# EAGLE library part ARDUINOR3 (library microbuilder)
This is a new object for the new Arduino R3 - with extra pins that you may want to use (such as IOref, and duplicated A4/A5
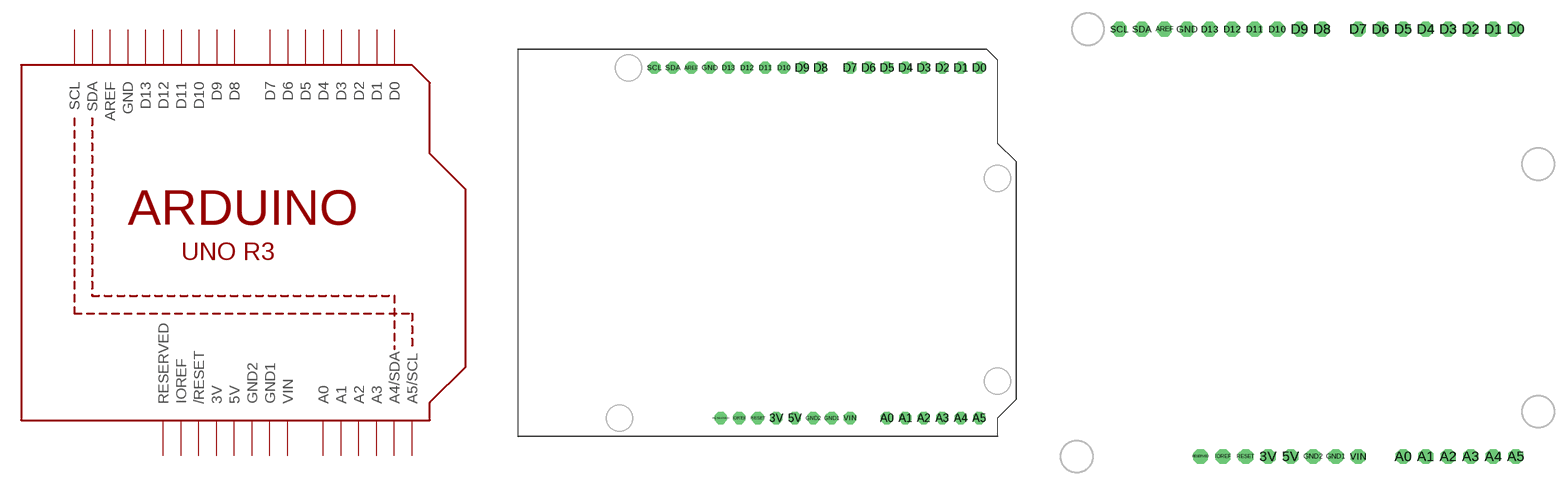
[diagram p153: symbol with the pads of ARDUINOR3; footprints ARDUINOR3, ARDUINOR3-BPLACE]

Designator prefix U

## ARDUINOR3-DIMENSION  [ARDUINOR3]
3V  3V  pwr
5V  5V  pwr
A0  A0
A1  A1
A2  A2
A3  A3
A4  A4/SDA
A5  A5/SCL
AREF  AREF
D0  D0
D1  D1
D2  D2
D3  D3
D4  D4
D5  D5
D6  D6
D7  D7
D8  D8
D9  D9
D10  D10
D11  D11
D12  D12
D13  D13
GND  GND  pwr
GND1  GND1  pwr
GND2  GND2  pwr
IOREF  IOREF  out
RESERVED  RESERVED  nc
RESET  /RESET
SCL  SCL
SDA  SDA
VIN  VIN  pwr

## ARDUINOR3-BPLACE  [ARDUINOR3-BPLACE]
Pads as for ARDUINOR3

## ARDUINOR3NODIM  [ARDUINOR3-NODIM]
Pads as for ARDUINOR3

## Footprint ARDUINOR3 (pad centres in mm)
The new Arduino R3 'classic' adds duplicate I2C pins and an IORef pin (and an unused pin
drill 1 pad 1.676 octagon: 3V 35.56,2.54; 5V 38.1,2.54; A0 50.8,2.54; A1 53.34,2.54; A2 55.88,2.54; A3 58.42,2.54; A4 60.96,2.54; A5 63.5,2.54; AREF 23.876,50.8; D0 63.5,50.8; D1 60.96,50.8; D2 58.42,50.8; D3 55.88,50.8; D4 53.34,50.8; D5 50.8,50.8; D6 48.26,50.8; D7 45.72,50.8; D8 41.656,50.8; D9 39.116,50.8; D10 36.576,50.8; D11 34.036,50.8; D12 31.496,50.8; D13 28.956,50.8; GND 26.416,50.8; GND1 43.18,2.54; GND2 40.64,2.54; IOREF 30.48,2.54; RESERVED 27.94,2.54; RESET 33.02,2.54; SCL 18.796,50.8; SDA 21.336,50.8; VIN 45.72,2.54

## Footprint ARDUINOR3-BPLACE (pad centres in mm)
drill 1 pad 1.676 octagon: 3V 35.56,2.54; 5V 38.1,2.54; A0 50.8,2.54; A1 53.34,2.54; A2 55.88,2.54; A3 58.42,2.54; A4 60.96,2.54; A5 63.5,2.54; AREF 23.876,50.8; D0 63.5,50.8; D1 60.96,50.8; D2 58.42,50.8; D3 55.88,50.8; D4 53.34,50.8; D5 50.8,50.8; D6 48.26,50.8; D7 45.72,50.8; D8 41.656,50.8; D9 39.116,50.8; D10 36.576,50.8; D11 34.036,50.8; D12 31.496,50.8; D13 28.956,50.8; GND 26.416,50.8; GND1 43.18,2.54; GND2 40.64,2.54; IOREF 30.48,2.54; RESERVED 27.94,2.54; RESET 33.02,2.54; SCL 18.796,50.8; SDA 21.336,50.8; VIN 45.72,2.54

## Footprint ARDUINOR3-NODIM (pad centres in mm)
drill 1 pad 1.676 octagon: 3V 35.56,2.54; 5V 38.1,2.54; A0 50.8,2.54; A1 53.34,2.54; A2 55.88,2.54; A3 58.42,2.54; A4 60.96,2.54; A5 63.5,2.54; AREF 23.876,50.8; D0 63.5,50.8; D1 60.96,50.8; D2 58.42,50.8; D3 55.88,50.8; D4 53.34,50.8; D5 50.8,50.8; D6 48.26,50.8; D7 45.72,50.8; D8 41.656,50.8; D9 39.116,50.8; D10 36.576,50.8; D11 34.036,50.8; D12 31.496,50.8; D13 28.956,50.8; GND 26.416,50.8; GND1 43.18,2.54; GND2 40.64,2.54; IOREF 30.48,2.54; RESERVED 27.94,2.54; RESET 33.02,2.54; SCL 18.796,50.8; SDA 21.336,50.8; VIN 45.72,2.54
